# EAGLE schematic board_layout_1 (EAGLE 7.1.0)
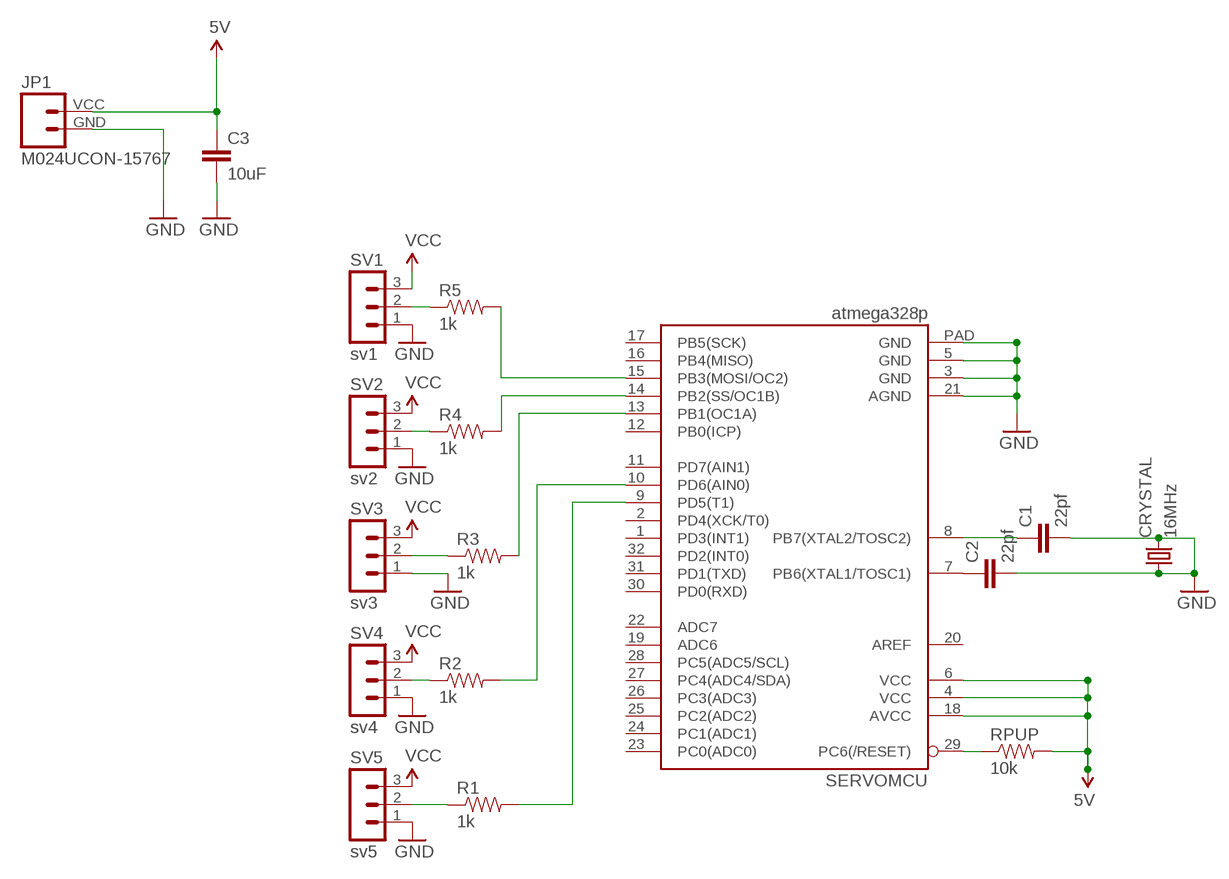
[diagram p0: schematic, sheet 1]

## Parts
C1  22pf  CAP0402-CAP  [0402-CAP]
C2  22pf  CAP0402-CAP  [0402-CAP]
C3  10uF  CAP0805  [0805]
CRYSTAL  16MHz  CRYSTALTC26V  [TC26V]
JP1  M024UCON-15767  [JST-2-SMD-VERT]
R1  1k  RESISTOR0402-RES  [0402-RES]
R2  1k  RESISTOR0402-RES  [0402-RES]
R3  1k  RESISTOR0402-RES  [0402-RES]
R4  1k  RESISTOR0402-RES  [0402-RES]
R5  1k  RESISTOR0402-RES  [0402-RES]
RPUP  10k  RESISTOR0402-RES  [0402-RES]
SERVOMCU  atmega328p  ATMEGA328P_MLFMLF32  [MLF32-PAD]
SV1  sv1  MA03-1  [MA03-1]
SV2  sv2  MA03-1  [MA03-1]
SV3  sv3  MA03-1  [MA03-1]
SV4  sv4  MA03-1  [MA03-1]
SV5  sv5  MA03-1  [MA03-1]

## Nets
GND: C1.2 C2.2 C3.2 CRYSTAL.1 CRYSTAL.2 JP1.GND SERVOMCU.3(GND) SERVOMCU.5(GND) SERVOMCU.21(AGND) SERVOMCU.PAD(GND) SV1.1 SV2.1 SV3.1 SV4.1 SV5.1
N$1: R5.2 SERVOMCU.15(PB3(MOSI/OC2))
N$2: R4.2 SERVOMCU.14(PB2(SS/OC1B))
N$3: R3.2 SERVOMCU.13(PB1(OC1A))
N$4: RPUP.1 SERVOMCU.29(PC6(/RESET))
N$5: R2.1 SV4.2
N$6: R1.1 SV5.2
N$7: R2.2 SERVOMCU.10(PD6(AIN0))
N$8: R1.2 SERVOMCU.9(PD5(T1))
N$9: R3.1 SV3.2
N$10: C1.1 SERVOMCU.8(PB7(XTAL2/TOSC2))
N$11: C2.1 SERVOMCU.7(PB6(XTAL1/TOSC1))
N$12: R5.1 SV1.2
N$13: R4.1 SV2.2
VCC: C3.1 JP1.VCC RPUP.2 SERVOMCU.4(VCC) SERVOMCU.6(VCC) SERVOMCU.18(AVCC) SV1.3 SV2.3 SV3.3 SV4.3 SV5.3 ; supply symbol labelled 5V
Unconnected: SERVOMCU.1(PD3(INT1)) SERVOMCU.2(PD4(XCK/T0)) SERVOMCU.11(PD7(AIN1)) SERVOMCU.12(PB0(ICP)) SERVOMCU.16(PB4(MISO)) SERVOMCU.17(PB5(SCK)) SERVOMCU.19(ADC6) SERVOMCU.20(AREF) SERVOMCU.22(ADC7) SERVOMCU.23(PC0(ADC0)) SERVOMCU.24(PC1(ADC1)) SERVOMCU.25(PC2(ADC2)) SERVOMCU.26(PC3(ADC3)) SERVOMCU.27(PC4(ADC4/SDA)) SERVOMCU.28(PC5(ADC5/SCL)) SERVOMCU.30(PD0(RXD)) SERVOMCU.31(PD1(TXD)) SERVOMCU.32(PD2(INT0))

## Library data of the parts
C1 C2 = SparkFun-Passives:CAP: Capacitor
C3 = SparkFun-Capacitors:CAP: Capacitor
CRYSTAL = crystal:CRYSTAL: CRYSTAL; OC_FARNELL: unknown; OC_NEWARK: unknown
JP1 = SparkFun-Connectors:M02: Standard 2-pin 0.1" header. Use with
R1-R5 RPUP = SparkFun-Passives:RESISTOR: Resistor
SERVOMCU = SparkFun-DigitalIC:ATMEGA328P_MLF: 32-Pin Atmega328 part Commonly used on Arduino compatible boards Available in QFP and QFN packages TQFP is IC-09069 QFN is non-stock
SV1-SV5 = con-lstb:MA03-1: PIN HEADER; OC_FARNELL: unknown; OC_NEWARK: unknown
